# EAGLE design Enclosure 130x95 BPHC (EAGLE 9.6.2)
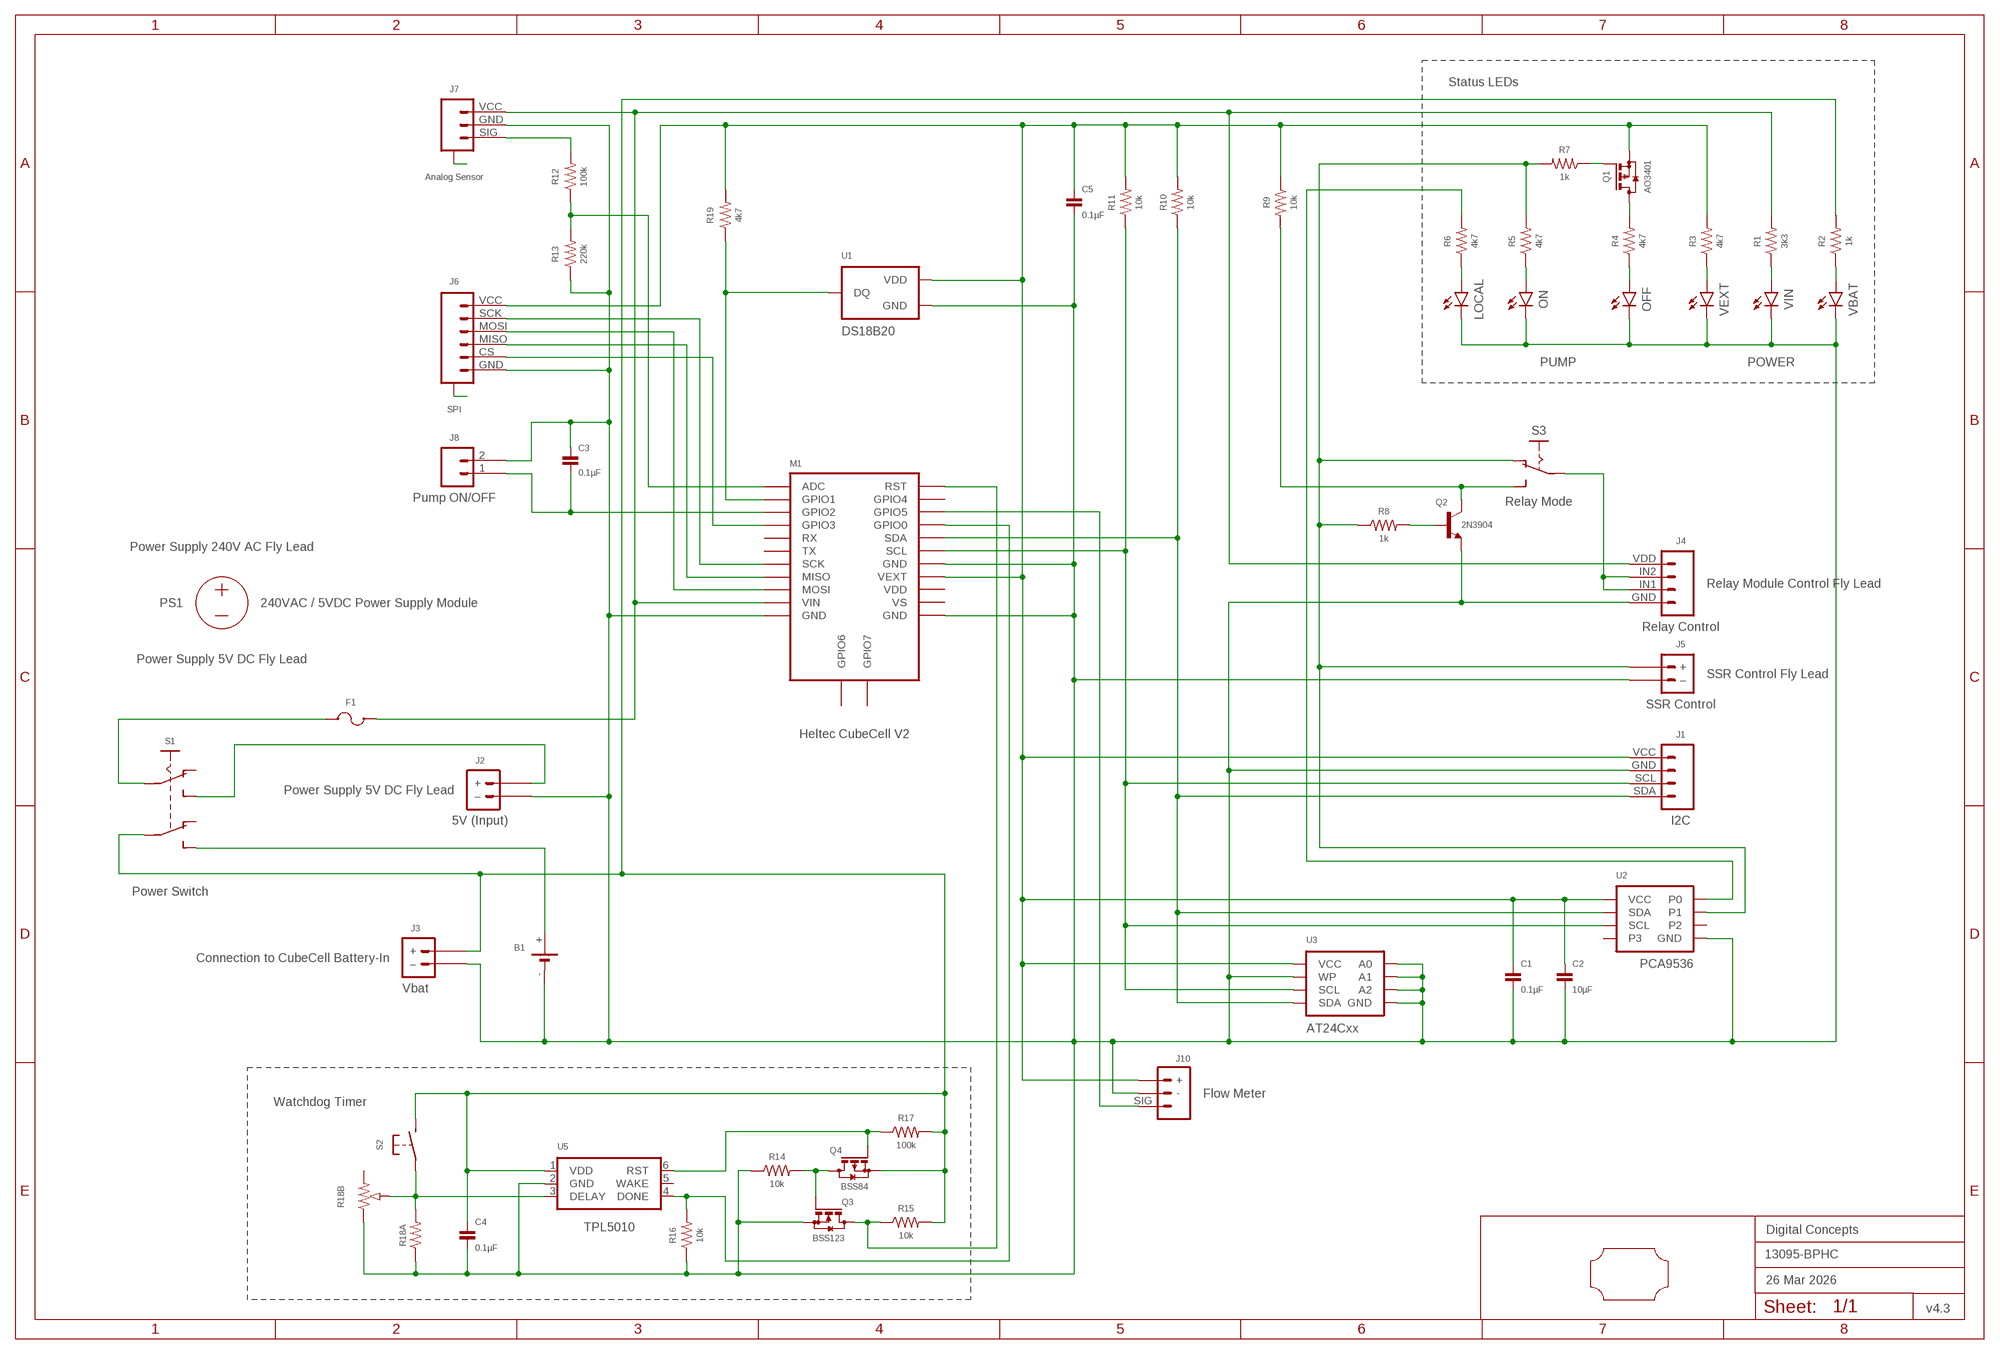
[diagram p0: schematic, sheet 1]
FRAME2 (A3L-LOC): DATE: 26 Mar 2026; OWNER: Digital Concepts; TITLE: 13095-BPHC; VERSION: v4.3

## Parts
B1  BATTERY-HOLDER-14500(AA)  [BATTERY-14500]
C1  0.1µF  CAPACITOR-0805  [C0805]
C2  10µF  CAPACITOR-0805  [C0805]
C3  0.1µF  CAPACITOR-0805  [C0805]
C4  0.1µF  CAPACITOR-0805  [C0805]
C5  0.1µF  CAPACITOR-0805  [C0805]
F1  Fuse  MF-PSMF050X-2  [F0805]
J1  I2C  HEADER-1X4-I2C  [CONN_04-I2C]
J2  5V (Input)  JST-PH2.0-2-VERTICAL-POWER  [JST-PH2.0-2-VERTICAL-POWER]
J3  Vbat  JST-GH1.25-2-HORIZONTAL-POWER  [JST-GH1.25-2-HORIZONTAL]
J4  Relay Control  JST-PH2.0-4-HORIZONTAL-RELAY  [JST-PH2.0-4-HORIZONTAL-RELAY]
J5  SSR Control  JST-PH2.0-2-H-POWER  [JST-PH2.0-2-HORIZONTAL-POWER]
J6  SPI  JST-SH1.0-6-SMD-HORIZONTAL-SPI  [JST-SH1.0-6-HORIZONTAL-SPI]
J7  Analog Sensor  JST-SH1.0-3-SMD-HORIZONTAL-SIG  [JST-SH1.0-3-HORIZONTAL-SIG]
J8  Pump ON/OFF  HEADER-1X2-GENERIC  [CONN_02-GENERIC]
J10  Flow Meter  JST-PH2.0-3-HORIZONTAL  [JST-PH2.0-3-HORIZONTAL-SIG]
LOCAL  LEDCHIP-LED0805  [CHIP-LED0805]
M1  Heltec CubeCell V2  HELTEC-CUBECELL  [HELTEC-CUBECELL]
OFF  LEDCHIP-LED0805  [CHIP-LED0805]
ON  LEDCHIP-LED0805  [CHIP-LED0805]
PCB1  PCB-OUTLINE-130X95-HALF-TOP  [PROTO-130X95-OUTLINE-HALF-TOP]
PS1  240VAC / 5VDC Power Supply Module  POWER_SUPPLY_MODULE  [AC_DC_POWER_SUPPLY]
Q1  AO3401  MOSFET-AO3401  [SOT-23]
Q2  2N3904  [SOT23-3]
Q3  BSS123  MOSFET-BSS123  [SOT23-3]
Q4  BSS84  MOSFET-BSS84  [SOT23-3]
R1  3k3  RESISTORR0805  [R0805]
R2  1k  RESISTORR0805  [R0805]
R3  4k7  RESISTORR0805  [R0805]
R4  4k7  RESISTORR0805  [R0805]
R5  4k7  RESISTORR0805  [R0805]
R6  4k7  RESISTORR0805  [R0805]
R7  1k  RESISTORR0805  [R0805]
R8  1k  RESISTOR-0805R0805  [R0805]
R9  10k  RESISTOR-0805R0805  [R0805]
R10  10k  RESISTORR0805  [R0805]
R11  10k  RESISTORR0805  [R0805]
R12  100k  RESISTORR0805  [R0805]
R13  220k  RESISTORR0805  [R0805]
R14  10k  RESISTORR0805  [R0805]
R15  10k  RESISTORR0805  [R0805]
R16  10k  RESISTORR0805  [R0805]
R17  100k  RESISTORR0805  [R0805]
R18A  RESISTORR0805  [R0805]
R18B  RESISTOR-TRIMM-33-US  [RTRIM3*3]
R19  4k7  RESISTORR0805  [R0805]
S1  Power Switch  SWITCH-SLIDE-DPDT-PTH  [SWITCH-DPDT-PTH]
S2  SWITCH-MOMENTARY-2-PIN  [SWITCH-2-PAD]
S3  Relay Mode  SWITCH-SLIDE-SPDT-SMT-R  [SWITCH-SPDT-SMT]
U1  DS18B20  THERMOMETER-DS18B20  [TO-92]
U2  PCA9536  PCA9536-I2C-GPIO4  [SOP-8]
U3  AT24Cxx  AT24CXX-EEPROM  [SOP-8]
U5  TPL5010  TPL5010DDCR  [SOT-23-6]
VBAT  LEDCHIP-LED0805  [CHIP-LED0805]
VEXT  LEDCHIP-LED0805  [CHIP-LED0805]
VIN  LEDCHIP-LED0805  [CHIP-LED0805]

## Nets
A6: J7.A@1(A) J7.A@3(A)
A8: J6.A@1(A) J6.A@6(A)
GND: B1.- C1.2 C2.2 C3.1 C4.2 C5.2 J1.GND J2.-(–) J3.-(–) J4.GND J5.-(–) J6.GND J7.GND J8.2 J10.- LOCAL.C M1.GND@11(GND) M1.GND@14(GND) M1.GND@18(GND) OFF.C ON.C Q2.2(E) Q3.2(S) R13.1 R14.1 R16.1 R18A.1 R18B.1(A) U1.1(GND) U2.4(GND) U3.1(A0) U3.2(A1) U3.3(A2) U3.4(GND) U3.7(WP) U5.2(GND) VBAT.C VEXT.C VIN.C
N$1: R6.2 U2.1(P0)
N$2: B1.+ S1.P$6(S2)
N$3: C3.2 J8.1 M1.GPIO2
N$4: Q2.1(B) R8.2
N$5: J1.SDA M1.SDA R10.1 U2.7(SDA) U3.5(SDA)
N$6: Q3.1(G) Q4.3(D) R14.2
N$8: M1.GPIO1 R19.1 U1.2(DQ)
N$9: J1.SCL M1.SCL R11.1 U2.6(SCL) U3.6(SCL)
N$10: R2.1 VBAT.A
N$11: M1.GPIO0 R16.2 U5.4(DONE)
N$12: OFF.A R4.1
N$13: R1.1 VIN.A
N$14: R3.1 VEXT.A
N$15: F1.2 S1.P$2(P1)
N$16: J2.+ S1.P$3(S1)
N$17: Q2.3(C) R9.2 S3.1(S)
N$18: M1.ADC R12.1 R13.2
N$19: ON.A R5.1
N$20: LOCAL.A R6.1
N$21: F1.1 J4.VDD J7.VCC M1.VIN R1.2
N$22: Q1.1(G) R7.1
N$23: Q1.3(D) R4.2
N$25: J7.SIG R12.2
N$26: J5.+ R5.2 R7.2 R8.1 S3.3(O) U2.2(P1)
N$27: J4.IN1 J4.IN2 S3.2(P)
N$28: J6.SCK M1.SCK
N$29: J6.MOSI M1.MOSI
N$30: J6.MISO M1.MISO
N$31: J6.CS M1.GPIO3
N$32: R18A.2 R18B.2(S) S2.P$1(P) U5.3(DELAY)
N$33: Q4.1(G) R17.1 U5.6(RST)
N$34: C4.1 J3.+ Q4.2(S) R2.2 R15.2 R17.2 S1.P$5(P2) S2.P$2(S) U5.1(VDD)
N$36: J10.SIG M1.GPIO5
N$37: M1.RST Q3.3(D) R15.1
VCC: C1.1 C2.1 C5.1 J1.VCC J6.VCC J10.+ M1.VEXT Q1.2(S) R3.2 R9.1 R10.2 R11.2 R19.2 U1.3(VDD) U2.8(VCC) U3.8(VCC)
Unconnected: M1.GPIO4 M1.GPIO6 M1.GPIO7 M1.RX M1.TX M1.VDD M1.VS R18B.3(E) S1.P$1(O1) S1.P$4(O2) U2.3(P2) U2.5(P3) U5.5(WAKE)

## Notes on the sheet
- Status LEDs
- PUMP | POWER
- Power Supply 240V AC Fly Lead
- Relay Module Control Fly Lead
- Power Supply 5V DC Fly Lead
- SSR Control Fly Lead
- Power Supply 5V DC Fly Lead
- Connection to CubeCell Battery-In
- Watchdog Timer

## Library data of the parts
B1 = digitalconcepts:BATTERY-HOLDER-14500(AA): 14500 (AA) battery holder
C1-C5 = digitalconcepts:CAPACITOR-0805: 0805 Capacitor
F1 = digitalconcepts:MF-PSMF050X-2: PTC Resettable Fuse
J1 = digitalconcepts:HEADER-1X4-I2C: I2C Interface [Pin 1 Vcc] 4-Pin Header
J2 = digitalconcepts:JST-PH2.0-2-VERTICAL-POWER: JST PH2.0 2P PTH Connector (Power)
J3 = digitalconcepts:JST-GH1.25-2-HORIZONTAL-POWER: JST GH1.25 2P PTH Connector (Power)
J4 = digitalconcepts:JST-PH2.0-4-HORIZONTAL-RELAY: PH2.0 4P Horizontal Connector with Relay Labels
J5 = digitalconcepts:JST-PH2.0-2-H-POWER: PH2.0 2P Right Angle Connector with power pin labelling
J6 = digitalconcepts:JST-SH1.0-6-SMD-HORIZONTAL-SPI: JST SH1.0 6P SMD SPI horizontal connector
J7 = digitalconcepts:JST-SH1.0-3-SMD-HORIZONTAL-SIG: JST SH1.0 3P SMD Horizontal Connector with Signal
J8 = digitalconcepts:HEADER-1X2-GENERIC: Single Row 2-Pin Header
J10 = digitalconcepts:JST-PH2.0-3-HORIZONTAL: PH2.0 3P Horizontal Connector
LOCAL OFF ON VBAT VEXT VIN = digitalconcepts:LED: LED
M1 = digitalconcepts:HELTEC-CUBECELL: Heltec CubeCell Development Board
PCB1 = digitalconcepts:PCB-OUTLINE-130X95-HALF-TOP: PCB half (sandwich top) enclosure (75 x 95) outline for 130 x 95 enclosure
PS1 = digitalconcepts:POWER_SUPPLY_MODULE: AC/DC Power Supply Module
Q1 = digitalconcepts:MOSFET-AO3401: AO3401 P-Channel MOSFET
Q2 = digitalconcepts:2N3904: 2N3904 NPN transistor
Q3 = digitalconcepts:MOSFET-BSS123: N-CHANNEL MOS FET
Q4 = digitalconcepts:MOSFET-BSS84: P-CHANNEL MOS FET
R1-R7 R10-R17 R18A R19 = digitalconcepts:RESISTOR: Resistor; SPICEPREFIX: R
R8 R9 = digitalconcepts:RESISTOR-0805: Resistor; SPICEPREFIX: R
R18B = digitalconcepts:RESISTOR-TRIMM-3*3-US: Trimm Resistor - 3*3 SMD
S1 = digitalconcepts:SWITCH-SLIDE-DPDT-PTH: Switch DPDT PTH
S2 = digitalconcepts:SWITCH-MOMENTARY-2-PIN: 2 Pin Momentary Switch
S3 = digitalconcepts:SWITCH-SLIDE-SPDT-SMT-R: Mini Sliding Switch SPDT SMT Reverse Polarity
U1 = digitalconcepts:THERMOMETER-DS18B20: Digital Thermometer -55C-125C TO92-3; AVAILABILITY: Bad; DESCRIPTION: Temperature Sensor Digital, Local -55°C ~ 125°C 12 b 8-uMAX; MF: Maxim Integrated; MP: DS18B20; PACKAGE: TO-92 Maxim Integrated; PRICE: None
U2 = digitalconcepts:PCA9536-I2C-GPIO4: PCA9536 4-bit I2C GPIO Expander
U3 = digitalconcepts:AT24CXX-EEPROM: AT24Cxx EEPROM SOP-8
U5 = digitalconcepts:TPL5010DDCR: TPL5010 Nano-Power System Timer with Watchdog

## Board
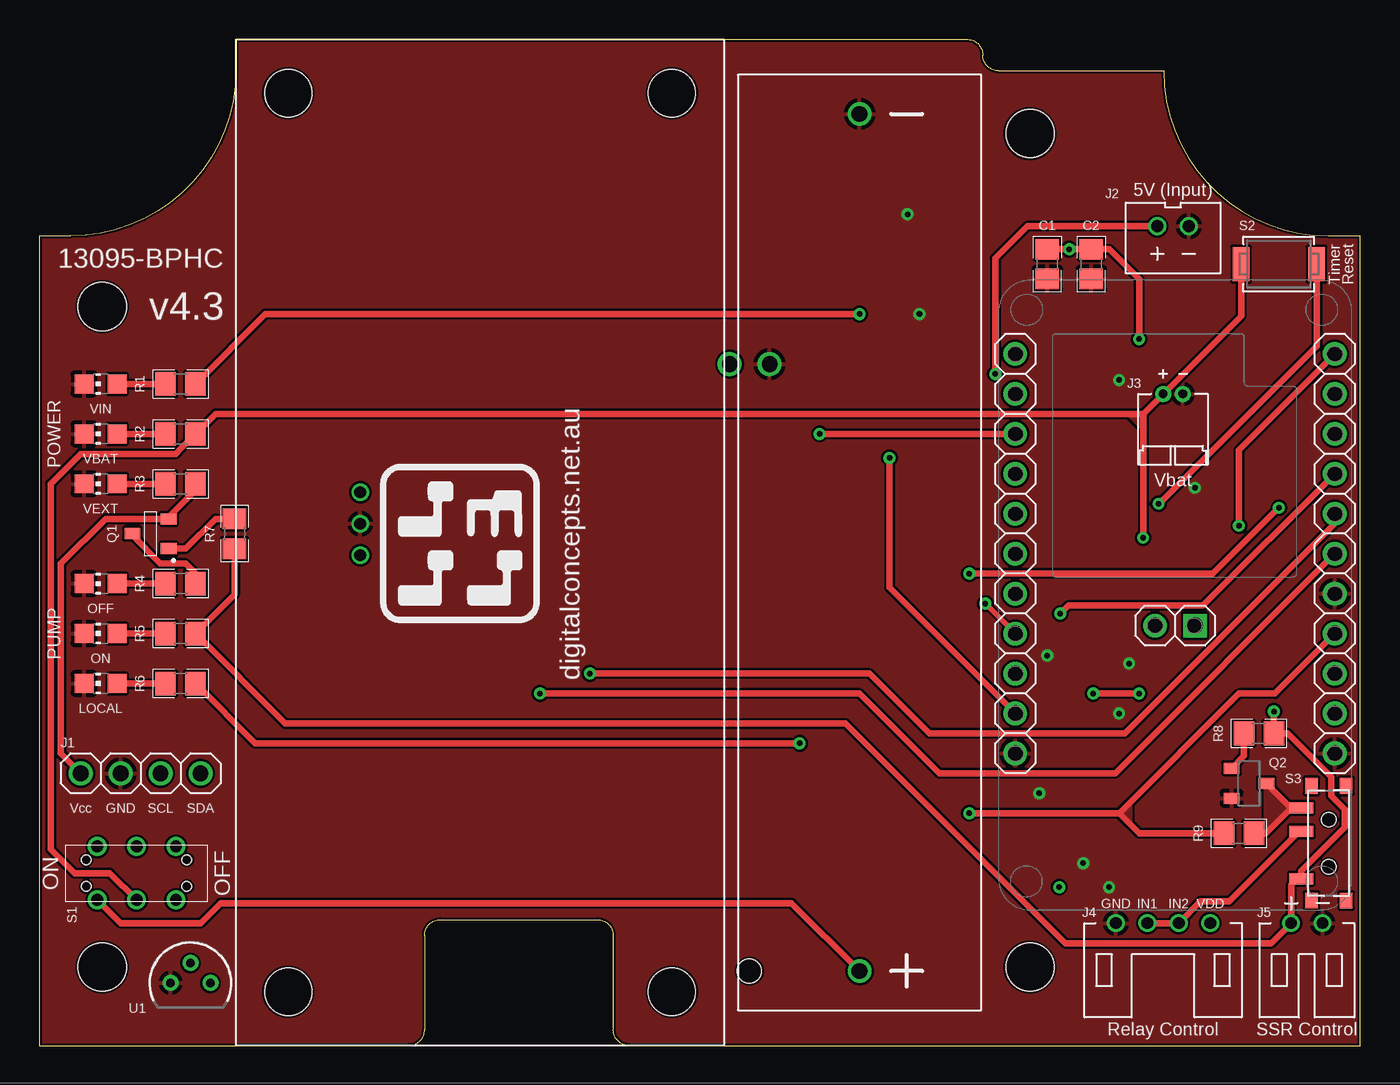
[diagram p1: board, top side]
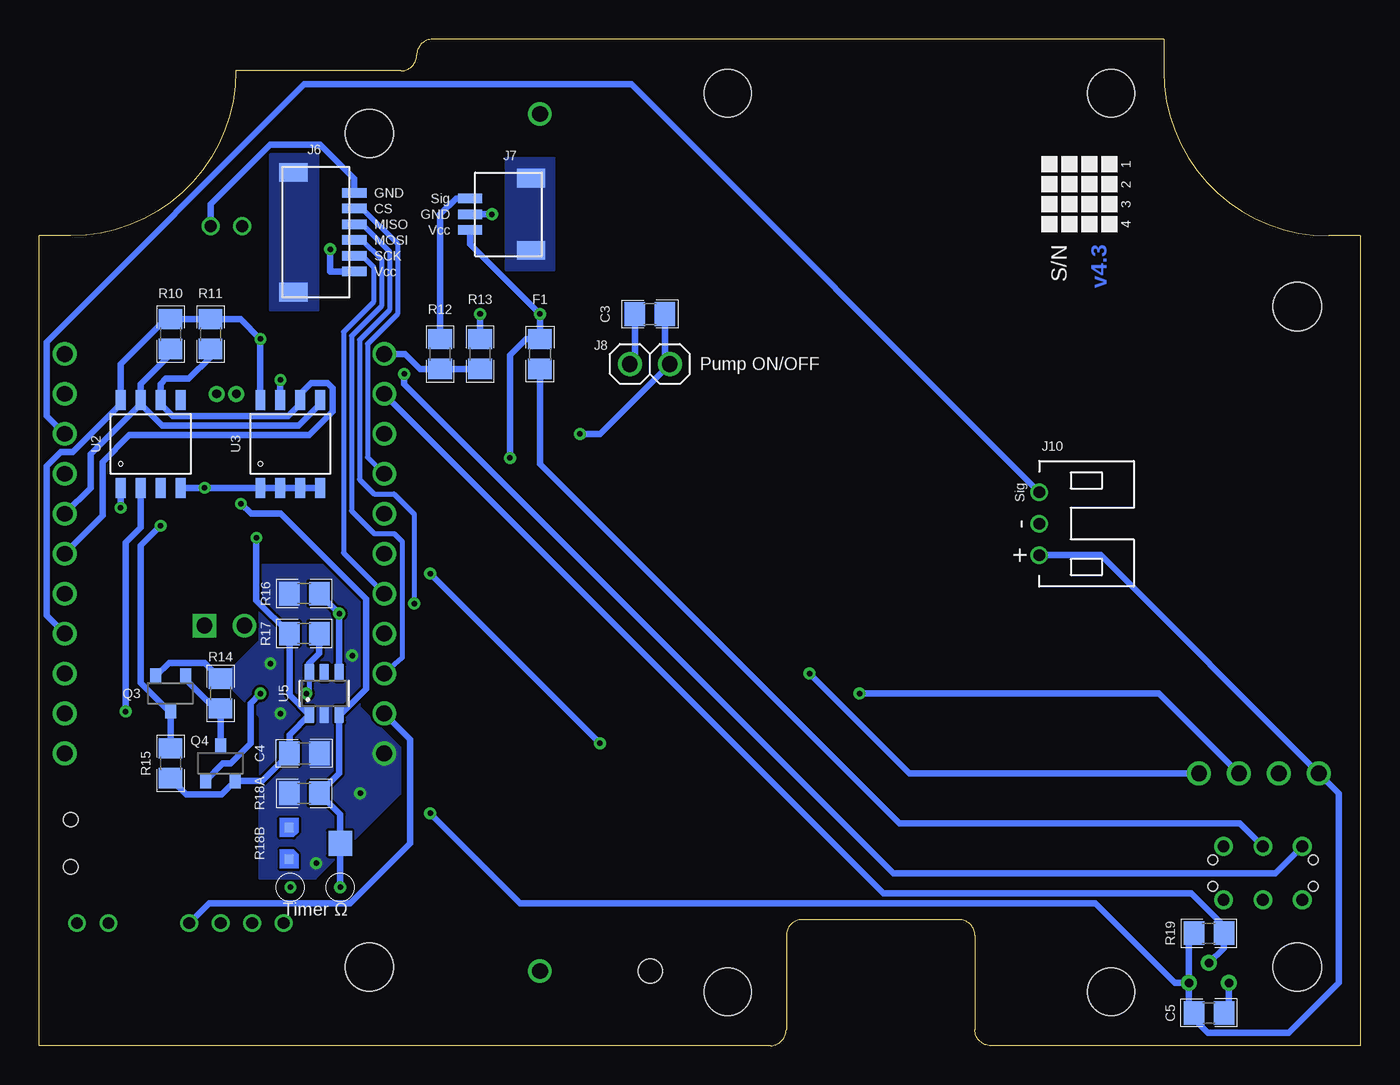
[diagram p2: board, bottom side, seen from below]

Size 84 x 64 mm. Coordinates in mm from the lower left corner, seen from the top.
Copper layers (1*16): Top 0.035mm / dielectric 1.5mm / Bottom 0.035mm
Design rules "default *": minimum track width 6mil, minimum drill 0.35mm, track to track 6mil, track to pad 6mil, pad to pad 6mil, via to via 6mil, smd to smd 6mil, copper to edge 6mil, drill to drill 6mil, minimum pad ring 1mil, minimum via ring 8mil, stop-mask expansion 4mil, vias tented up to drill 0mil, thermal gap 10mil

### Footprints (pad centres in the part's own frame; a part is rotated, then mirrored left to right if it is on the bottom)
BATTERY-14500 = drill 1: + -27.25,0; - 27.25,0 | hole 1.524: -27.25,7
C0805 = smd 1.3 x 1.5: 1 -0.95,0; 2 0.95,0
F0805 = smd 1.3 x 1.5: 1 -0.95,0; 2 0.95,0
CONN_04-I2C = drill 1 pad 1.524: GND 2.54,0; SCL 5.08,0; SDA 7.62,0; VCC 0,0
JST-PH2.0-2-VERTICAL-POWER = drill 0.75: + -1,0; - 1,0
JST-GH1.25-2-HORIZONTAL = drill 0.55 pad 1.016: + -0.625,0; - 0.625,0
JST-PH2.0-4-HORIZONTAL-RELAY = drill 0.75: GND 3,0; IN1 1,0; IN2 -1,0; VDD -3,0
JST-PH2.0-2-HORIZONTAL-POWER = drill 0.75: + 1,0; - -1,0
JST-SH1.0-6-HORIZONTAL-SPI = smd 1.2 x 1.8: A@1 -3.8,-1.335; A@6 3.8,-1.335 | smd 0.6 x 1.55: CS -1.5,2.54; GND -2.5,2.54; MISO -0.5,2.54; MOSI 0.5,2.54; SCK 1.5,2.54; VCC 2.5,2.54
JST-SH1.0-3-HORIZONTAL-SIG = smd 1.2 x 1.8: A@1 -2.3,-1.335; A@3 2.3,-1.335 | smd 0.6 x 1.55: GND 0,2.54; SIG 1,2.54; VCC -1,2.54
CONN_02-GENERIC = drill 1 pad 1.524: 1 0,0; 2 2.54,0
JST-PH2.0-3-HORIZONTAL-SIG = drill 0.75: + 2,0; - 0,0; SIG -2,0
CHIP-LED0805 = smd 1.2 x 1.2: A 0,-1.05; C 0,1.05
HELTEC-CUBECELL = drill 1: ADC 0,0; GND@11 0,25.4; GND@14 -20.32,25.4; GND@18 -20.32,15.24; GPIO0 -20.32,7.62; GPIO1 0,2.54; GPIO2 0,5.08; GPIO3 0,7.62; GPIO4 -20.32,2.54; GPIO5 -20.32,5.08; GPIO6 -8.89,17.272; MISO 0,17.78; MOSI 0,20.32; RST -20.32,0; RX 0,10.16; SCK 0,15.24; SCL -20.32,12.7; SDA -20.32,10.16; TX 0,12.7; VDD -20.32,20.32; VEXT -20.32,17.78; VIN 0,22.86; VS -20.32,22.86 | drill 1 square: GPIO7 -11.43,17.272
PROTO-130X95-OUTLINE-HALF-TOP = hole 3.048: -38,10; 21,21; 21,-32; -38,-32
AC_DC_POWER_SUPPLY = hole 3: -28.575,12.192; -28.575,-12.192; 28.575,-12.192; 28.575,12.192
SOT-23 = smd 0.7 x 1: 1 -0.95,-1.15; 2 0.95,-1.15; 3 0,1.15
SOT23-3 = smd 0.7 x 1: 1 -0.95,-1.1; 2 0.95,-1.1; 3 0,1.1
R0805 = smd 1.3 x 1.5: 1 -0.95,0; 2 0.95,0
RTRIM3*3 = smd 0.6 x 0.6: 1 -1,-1.6; 3 1,-1.6 | smd 1.6 x 1.5: 2 0,1.65
SWITCH-DPDT-PTH = drill 0.75 pad 1.19: P$1 -1.7,2.5; P$2 -1.7,0; P$3 -1.7,-2.5; P$4 1.7,2.5; P$5 1.7,0; P$6 1.7,-2.5 | hole 0.6: 0.85,3.2; -0.85,3.2; 0.85,-3.2; -0.85,-3.2
SWITCH-2-PAD = smd 1.067 x 2.184: P$1 -2.4,0; P$2 2.4,0
SWITCH-SPDT-SMT = smd 0.7 x 1.5: 1 2.25,1.75; 2 0.75,1.75; 3 -2.25,1.75 | smd 1 x 0.8: GND@1 3.65,-1.1; GND@2 3.65,1.1; GND@3 -3.65,1.1; GND@4 -3.65,-1.1 | hole 0.9: -1.5,0; 1.5,0
TO-92 = drill 0.55 pad 1.016: 1 -1.27,0; 2 0,1.27; 3 1.27,0
SOP-8 = smd 0.635 x 1.27: 1 -1.905,-2.794; 2 -0.635,-2.794; 3 0.635,-2.794; 4 1.905,-2.794; 5 1.905,2.794; 6 0.635,2.794; 7 -0.635,2.794; 8 -1.905,2.794
SOT-23-6 = smd 1.1 x 0.6: 1 -1.35,0.95; 2 -1.35,0; 3 -1.35,-0.95; 4 1.35,-0.95; 5 1.35,0; 6 1.35,0.95

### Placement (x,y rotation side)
B1  52.16,32 90 top
C1  64.1,49.7 270 top
C2  66.89,49.7 270 top
C3  45.17,46.53 0 bottom
C4  67.15,18.59 0 bottom
C5  9.61,2.08 0 bottom
F1  52.16,43.98 270 bottom
J1  2.63,17.32 0 top
J2  72.1,52.11 0 top
J3  72.1,41.45 0 top
J4  71.46,7.79 180 top
J5  80.61,7.79 180 top
J6  66.51,51.73 270 bottom
J7  54.06,52.88 90 bottom
J8  43.91,43.35 180 bottom
J10  20.41,33.19 270 bottom
LOCAL  3.9,23.03 90 top
M1  62.07,43.98 180 top
OFF  3.9,29.38 90 top
ON  3.9,26.21 90 top
PCB1  42,37 0 top
PS1  28.03,32 90 top
Q1  7.07,32.55 90 top
Q2  76.92,16.68 270 top
Q3  75.66,22.4 180 bottom
Q4  72.48,17.95 0 bottom
R1  8.98,42.08 0 top
R2  8.98,38.91 0 top
R3  8.98,35.73 0 top
R4  8.98,29.38 0 top
R5  8.98,26.21 0 top
R6  8.98,23.03 0 top
R7  12.41,32.55 270 top
R8  77.56,19.86 180 top
R9  76.29,13.51 0 top
R10  75.66,45.26 90 bottom
R11  73.11,45.26 90 bottom
R12  58.51,43.98 90 bottom
R13  55.97,43.98 270 bottom
R14  72.48,22.4 270 bottom
R15  75.66,17.95 270 bottom
R16  67.15,28.75 0 bottom
R17  67.15,26.21 180 bottom
R18A  67.15,16.05 0 bottom
R18B  66.51,12.87 270 bottom
R19  9.61,7.16 180 bottom
S1  6.19,10.97 270 top
S2  78.83,49.7 180 top
S3  82,12.87 90 top
U1  9.61,3.98 0 top
U2  76.92,38.27 0 bottom
U3  68.03,38.27 0 bottom
U5  65.88,22.4 90 bottom
VBAT  3.9,38.91 90 top
VEXT  3.9,35.73 90 top
VIN  3.9,42.08 90 top

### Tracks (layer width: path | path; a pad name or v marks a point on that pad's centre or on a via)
A6
  pour Bottom (no thermals): 51.27,56.43 54.32,56.43 54.32,49.32 51.27,49.32
A8
  pour Bottom (no thermals): 69.3,56.69 69.3,46.78 66.26,46.78 66.26,56.69
GND  (via drill 0.35)
  Bottom 0.406: U3.4 U3.3 U3.2 U3.1 v73.5,35.48 U2.4 | C3.1 46.12,43.67 J8.2 | J2.- 73.1,53.51 69.32,57.29 66.14,57.29 63.97,55.12 J6.GND | v55.21,52.88 J7.GND | R13.1 v55.97,46.53 | U1.1 8.34,2.4 C5.2 | U3.7 v68.67,42.33 | Q3.2 75.75,24.35 73.49,24.35 R14.1
  other vias: 68.03,10.08 68.67,21.13 66.38,11.6 63.59,16.05 64.1,24.81 69.3,24.3
  pour Top (rank 5): -1.18,64.94 -1.18,-1.1 85.18,-1.1 85.18,64.94
  pour Bottom (rank 2, no thermals): 69.98,30.57 69.98,25.78 71.84,23.92 71.84,22.78 69.95,20.88 69.98,10.63 66.43,10.63 61.05,16 61.05,18.97 63.63,21.55 63.63,30.57
N$1  (via drill 0.35)
  Top 0.406: v48.35,19.22 13.74,19.22 R6.2 | v78.83,34.21 74.64,30.02 v59.14,30.02
  Bottom 0.406: v59.14,30.02 v48.35,19.22 | U2.1 v78.83,34.21
N$2
  Top 0.406: B1.+ 47.85,9.06 11.52,9.06 10.25,7.79 5.16,7.79 S1.P$6
N$3  (via drill 0.35)
  Top 0.406: M1.GPIO2 v49.62,38.91
  Bottom 0.406: v49.62,38.91 48.35,38.91 J8.1 44.23,43.67 C3.2
N$4
  Top 0.406: R8.2 76.61,18.42 Q2.1
N$5  (via drill 0.35)
  Top 0.406: M1.SDA 82.39,33.22 69.02,19.86 56.61,19.86 52.8,23.67 v35.02,23.67
  Bottom 0.406: v35.02,23.67 28.66,17.32 J1.SDA | R10.1 75.66,43.98 77.56,42.08 U2.7 77.56,40.81 | 77.56,40.81 80.73,37.64 80.73,35.48 M1.SDA | U3.5 66.13,40.81 67.5,39.44 76.19,39.44 77.56,40.81
N$6
  Bottom 0.406: Q4.3 R14.2 72.86,21.45 74.7,23.29 Q3.1
N$8
  Bottom 0.406: U1.2 8.66,6.2 R19.1 8.66,7.61 10.75,9.7 30.32,9.7 M1.GPIO1
N$9  (via drill 0.35)
  Top 0.406: M1.SCL 68.42,17.32 57.24,17.32 52.16,22.4 v31.84,22.4
  Bottom 0.406: J1.SCL 12.79,22.4 v31.84,22.4 | M1.SCL 79.97,33.7 79.97,37.13 78.27,38.83 66.84,38.83 65.36,40.32 65.36,41.81 65.67,42.12 66.72,42.12 67.4,41.45 U3.6 67.4,40.81 68.16,40.05 75.53,40.05 76.29,40.81 U2.6 76.29,42.08 75.96,42.41 74.5,42.41 73.11,43.8 R11.1
N$10
  Top 0.406: VBAT.A 6.44,38.91 R2.1
N$11  (via drill 0.35)
  Top 0.406: M1.GPIO0 74,27.98 65.43,27.98 v64.92,27.48
  Bottom 0.406: U5.4 v64.92,27.48 R16.2
N$12
  Top 0.406: R4.1 6.44,29.38 OFF.A
N$13
  Top 0.406: VIN.A 6.44,42.08 R1.1
N$14
  Top 0.406: R3.1 6.44,35.73 VEXT.A
N$15
  Bottom 0.406: F1.2 52.16,37 29.3,14.14 7.66,14.14 S1.P$2
N$16  (via drill 0.35)
  Top 0.406: v60.8,42.72 60.8,50.08 62.83,52.11 J2.+
  Bottom 0.406: v60.8,42.72 60.8,42.08 29.68,10.97 5.39,10.97 S1.P$3
N$17
  Top 0.406: R9.2 78,13.51 79.58,15.09 79.58,15.12 | S3.1 79.58,15.12 | 79.58,15.12 Q2.3
  pour Top (no thermals): 79.66,15.22 77.94,16.93 77.94,13.51
N$18
  Bottom 0.406: R13.2 R12.1 59.78,43.04 60.73,43.98 M1.ADC
N$19
  Top 0.406: R5.1 6.44,26.21 ON.A
N$20
  Top 0.406: LOCAL.A 6.44,23.03 R6.1
N$21  (via drill 0.35)
  Top 0.406: v52.16,46.53 14.38,46.53 R1.2 | v54.06,37.38 54.06,29.13 M1.VIN
  Bottom 0.406: v54.06,37.38 54.06,43.92 53.05,44.94 F1.1 v52.16,46.53 56.61,50.97 J7.VCC | M1.VIN 60.41,19.47 60.41,12.87 64.22,9.06 73.19,9.06 J4.VDD
N$22
  Top 0.406: Q1.1 9.3,31.61 11.2,33.51 R7.1
N$23
  Top 0.406: R4.2 9.93,30.02 9.29,30.65 7.7,30.65 5.92,32.43 Q1.3
N$25
  Bottom 0.406: J7.SIG 57.51,53.88 58.51,52.88 R12.2
N$26  (via drill 0.35)
  Top 0.406: R7.2 12.41,28.68 R5.2 15.64,20.49 51.27,20.49 65.24,6.52 78.34,6.52 J5.+ 79.61,10.22 80.01,10.62 S3.3 80.25,11.12 83.02,13.89 83.02,15.03 82.16,15.89 82.16,17.09 79.39,19.86 R8.1 v78.51,21.25
  Bottom 0.406: U2.2 77.56,32.94 78.51,31.99 v78.51,21.25
N$27
  Top 0.406: J4.IN1 J4.IN2 73.85,9.18 75.68,9.18 80.13,13.62 S3.2
N$28
  Bottom 0.305: J6.SCK 63.46,50.23 62.75,49.52 62.75,47.29 64.66,45.38 64.66,31.34 M1.SCK
N$29
  Bottom 0.305: J6.MOSI 63.46,51.23 62.24,50.01 62.24,47.03 64.15,45.13 64.15,34 62.7,32.55 61.43,32.55 60.92,32.05 60.92,24.66 M1.MOSI
N$30  (via drill 0.35)
  Top 0.305: M1.MISO v60.16,28.11
  Bottom 0.305: J6.MISO 63.46,52.23 61.74,50.51 61.74,46.78 63.64,44.87 63.64,36.01 62.71,35.08 61.44,35.08 60.16,33.8 v60.16,28.11
N$31
  Bottom 0.305: M1.GPIO3 63.13,37.43 63.13,44.62 61.23,46.53 61.23,51 63.46,53.23 J6.CS
N$32  (via drill 0.35)
  Top 0.406: S2.P$1 81.23,44.48 71.21,34.46 v71.18,34.46
  Bottom 0.406: v64.86,10.08 R18B.2 64.86,14.71 R18A.2 64.93,17.32 U5.3 64.86,21.05 63.21,22.7 63.21,28.4 68.64,33.83 70.54,33.83 v71.18,34.46
N$33  (via drill 0.35)
  Top 0.406: v69.94,22.4 v67.02,22.4
  Bottom 0.305: v67.02,22.4 66.83,22.59 U5.6
  Bottom 0.406: U5.6 66.83,24.31 66.2,24.94 R17.1 | Q4.1 72.33,17.95 71.84,17.95 70.58,19.22 70.58,21.76 v69.94,22.4
N$34  (via drill 0.35)
  Top 0.406: S1.P$5 4.49,10.97 2.25,10.97 0.72,12.49 0.72,35.73 2.63,37.64 8.66,37.64 9.04,38.01 R2.2 11.2,40.18 70.19,40.18 | 70.19,40.18 J3.+ 76.43,46.4 S2.P$2 | 70.19,40.18 v70.19,32.3
  Bottom 0.406: R15.2 74.64,15.99 72.39,15.99 Q4.2 69.83,16.85 C4.1 68.1,19.78 U5.1 68.1,22.32 R17.2 70.19,28.3 v70.19,32.3
  pour Top (no thermals): 70.19,40.18 69.3,40.18 70.19,39.29
N$36
  Bottom 0.406: J10.SIG 46.35,61.13 67.15,61.13 83.53,44.75 83.53,40.05 M1.GPIO5
N$37  (via drill 0.35)
  Top 0.406: M1.RST 76.29,37.89 v76.29,33.06
  Bottom 0.406: R15.1 Q3.3 75.78,21.3 77.56,23.07 77.56,31.79 v76.29,33.06
VCC  (via drill 0.35, 0.35 pad 0.55)
  Top 0.406: J1.VCC 1.36,18.59 1.36,30.65 4.21,33.51 Q1.2 8.22,33.63 9.93,35.34 R3.2 | M1.VEXT 78.58,22.4 76.29,22.4 68.67,14.78 | 68.67,14.78 v59.14,14.78 | v69.94,44.94 69.94,48.75 68.03,50.65 C2.1 v65.5,50.65 C1.1 | R9.1 69.94,13.51 68.67,14.78
  Bottom 0.406: v59.14,14.78 53.43,9.06 16.86,9.06 11.77,3.98 U1.3 | M1.VEXT 83.53,27.35 83.53,36.87 82.64,37.76 81.88,37.76 78.83,40.81 U2.8 78.83,43.35 75.97,46.21 R10.2 R11.2 71.21,46.21 v69.94,44.94 U3.8 | J10.+ 16.5,31.19 J1.VCC 1.36,16.05 1.36,3.98 4.53,0.81 9.68,0.81 10.56,1.69 C5.1 10.88,2.4 U1.3 | R19.2 10.88,6.84 U1.3 | v65.5,50.65 65.5,49.23 J6.VCC
  pour Top (no thermals): 68.67,14.78 69.3,15.41 69.3,14.14

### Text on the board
Bottom: v4.3
tPlace: 13095-BPHC | digitalconcepts.net.au
bPlace: 1 | 2 | 3 | 4 | S/N
tNames: Timer / Reset | v4.3 | POWER | PUMP | Vcc | GND | SCL | SDA | ON | OFF
bNames: GND | Sig | CS | GND | MISO | Vcc | MOSI | SCK | Vcc | Timer Ω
